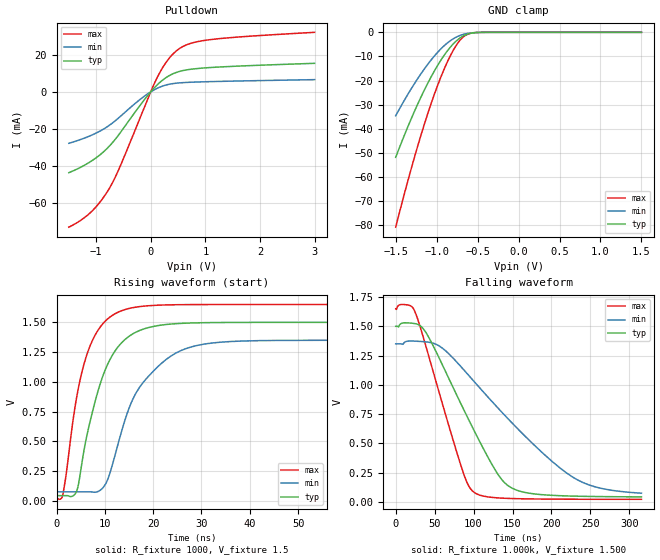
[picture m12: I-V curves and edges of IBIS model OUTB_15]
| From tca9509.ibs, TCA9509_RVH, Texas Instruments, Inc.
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[Model]   OUTB_15
Model_type  Open_drain
Enable   Active-High
Vref =   1.5
Rref =   1350
Cref =   50p
Vmeas =   0.75
| variable   typ   min   max
C_comp   2.63pF   1.78pF   3.10pF
| C_pulldown   3.02pF   2.10pF   4.29pF
| C_tri-state   2.63pF   1.78pF   3.10pF
[Temperature Range]   40   100   -40
| Ambient temperature   25   85   -40
[Voltage range]   1.5   1.35   1.65
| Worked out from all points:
|   slope of the pulldown table from 0 to 0.225 V, typ, clamps not added: 34.6 ohm
|   GND clamp passes 1 mA (typ) near -0.64 V on its own axis
|   rising waveform, R_fixture 1000, V_fixture 1.5: 20-80 % time 6.03ns typ, 8.43ns min, 4.79ns max; typ from 0.043 V to 1.5 V
|   falling waveform, R_fixture 1.000k, V_fixture 1.500: 20-80 % time 65.1ns typ, 112ns min, 43ns max; typ from 1.5 V to 0.044 V
[GND Clamp]
| OUTB_15
|   Voltage   I(typ)   I(min)   I(max)
-1.5V     -51.84mA   -34.6mA    -80.81mA
-1.37V    -40.68mA   -26.78mA   -63.94mA
-1.25V    -31.18mA   -20.17mA   -49.37mA
-1.135V   -22.9mA    -14.48mA   -36.51mA
-1.03V    -16.16mA   -9.92mA    -25.9mA
-930mV    -10.6mA    -6.259mA   -17mA
-835mV    -6.238mA   -3.535mA   -9.876mA
-750mV    -3.277mA   -1.815mA   -4.87mA
-670mV    -1.422mA   -812.2uA   -1.79mA
-595mV    -490.4uA   -316.4uA   -474.2uA
-480mV    -58.09uA   -51.13uA   -33.15uA
1.5V      328.8pA    1.515nA    103.4pA
[Pulldown]
| OUTB_15
|   Voltage   I(typ)   I(min)   I(max)
-1.5V     -43.71mA   -27.83mA   -73.16mA
-1.1V     -37.68mA   -23.65mA   -65.17mA
-930mV    -34.08mA   -21.23mA   -59.62mA
-775mV    -29.87mA   -18.44mA   -53.03mA
-570mV    -22.58mA   -13.65mA   -40.93mA
-160mV    -5.939mA   -3.312mA   -11.55mA
110mV     3.531mA    1.79mA     7.22mA
290mV     7.87mA     3.753mA    16.3mA
480mV     10.6mA     4.708mA    22.39mA
705mV     12.08mA    5.14mA     25.94mA
1.055V    13.06mA    5.482mA    28.08mA
3V        15.41mA    6.586mA    32.16mA
[Ramp]
| OUTB_15
| variable   typ   min   max
dV/dt_r   0.88/6.03E-09   0.77/8.42E-09   0.98/4.78E-09
dV/dt_f   0.89/6.64E-08   0.77/1.14E-07   1.00/4.39E-08
R_load = 1000
[Rising Waveform]
| OUTB_15
R_fixture =   1000
C_fixture =   0
L_fixture =   0
V_fixture =   1.5
V_fixture_min = 1.35
V_fixture_max = 1.65
|   Time   V(typ)   V(min)   V(max)
0s        42.93mV    75.33mV    23.16mV
1.349ns   42.92mV    75.33mV    59.26mV
4.165ns   81mV       75.33mV    869.2mV
7.045ns   683.7mV    75.18mV    1.312V
9.605ns   1.051V     109.4mV    1.489V
11.46ns   1.217V     288mV      1.556V
17.22ns   1.432V     956.1mV    1.633V
25.67ns   1.491V     1.261V     1.649V
38.4ns    1.499V     1.343V     1.65V
315.6ns   1.5V       1.35V      1.65V
[Falling Waveform]
R_fixture = 1.000k
V_fixture = 1.500
V_fixture_min = 1.350
V_fixture_max = 1.650
C_fixture = 0.000
L_fixture = 0.000
|  time   V(typ)   V(min)   V(max)
0s        1.5V       1.35V      1.65V
14.53ns   1.529V     1.372V     1.683V
24.64ns   1.523V     1.373V     1.626V
41.22ns   1.42V      1.365V     1.274V
84.81ns   824.3mV    1.148V     290.6mV
100.3ns   615.4mV    1.032V     85.03mV
132.6ns   224mV      793.3mV    35.02mV
153.8ns   105.4mV    645mV      29.28mV
234.1ns   49.89mV    187.3mV    24.06mV
315.6ns   44.42mV    75.44mV    23.32mV
